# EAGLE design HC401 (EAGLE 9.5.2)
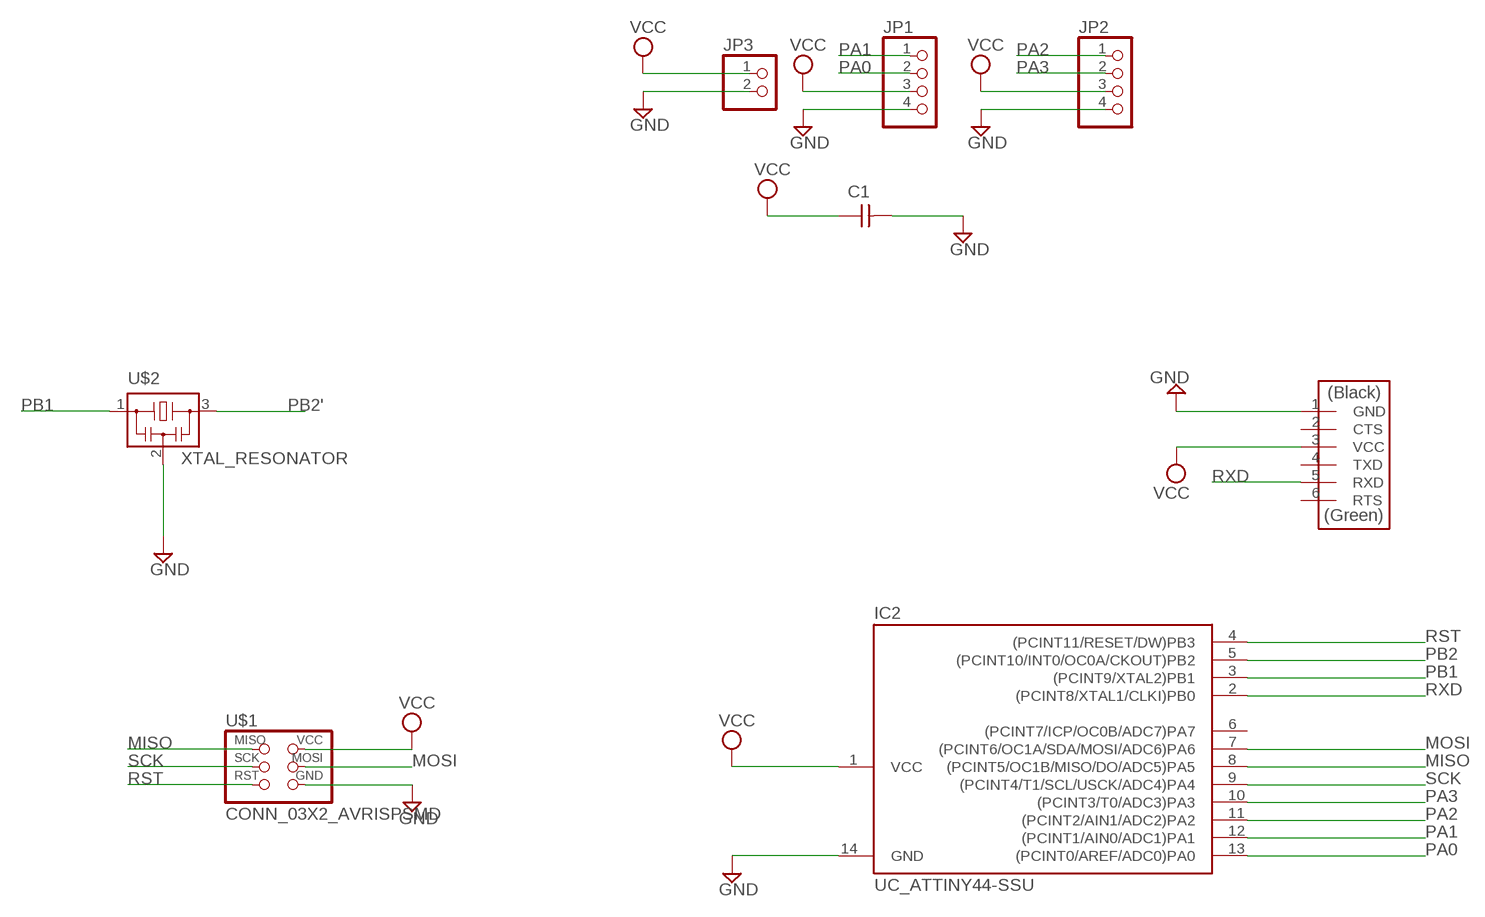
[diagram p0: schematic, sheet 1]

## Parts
C1  CAP_UNPOLARIZED  [C1206]
IC2  UC_ATTINY44-SSU  [SOIC14]
JP1  PINHD-1X4  [1X04]
JP2  PINHD-1X4  [1X04]
JP3  PINHD-1X2  [1X02]
U$1  CONN_03X2_AVRISPSMD  [2X03SMD]
U$2  XTAL_RESONATOR  [EFOBM]
U$3  CONN_06_FTDI-SMD-HEADER  [1X06SMD]

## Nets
GND: C1.2 IC2.14(GND) JP1.4 JP2.4 JP3.2 U$1.6(GND) U$2.2 U$3.1(GND)
MISO: IC2.8((PCINT5/OC1B/MISO/DO/ADC5)PA5) U$1.1(MISO)
MOSI: IC2.7((PCINT6/OC1A/SDA/MOSI/ADC6)PA6) U$1.4(MOSI)
PA0: IC2.13((PCINT0/AREF/ADC0)PA0) JP1.2
PA1: IC2.12((PCINT1/AIN0/ADC1)PA1) JP1.1
PA2: IC2.11((PCINT2/AIN1/ADC2)PA2) JP2.1
PA3: IC2.10((PCINT3/T0/ADC3)PA3) JP2.2
PB1: IC2.3((PCINT9/XTAL2)PB1) U$2.1
PB2: IC2.5((PCINT10/INT0/OC0A/CKOUT)PB2)
PB2': U$2.3
RST: IC2.4((PCINT11/RESET/DW)PB3) U$1.5(RST)
RXD: IC2.2((PCINT8/XTAL1/CLKI)PB0) U$3.5(RXD)
SCK: IC2.9((PCINT4/T1/SCL/USCK/ADC4)PA4) U$1.3(SCK)
VCC: C1.1 IC2.1(VCC) JP1.3 JP2.3 JP3.1 U$1.2(VCC) U$3.3(VCC)
Unconnected: IC2.6((PCINT7/ICP/OC0B/ADC7)PA7) U$3.2(CTS) U$3.4(TXD) U$3.6(RTS)

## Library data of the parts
C1 = fab:CAP_UNPOLARIZED
IC2 = fab:UC_ATTINY44
JP1 JP2 = pinhead:PINHD-1X4: PIN HEADER
JP3 = pinhead:PINHD-1X2: PIN HEADER
U$1 = fab:CONN_03X2_AVRISP
U$2 = fab:XTAL_RESONATOR
U$3 = fab:CONN_06_FTDI-SMD-HEADER

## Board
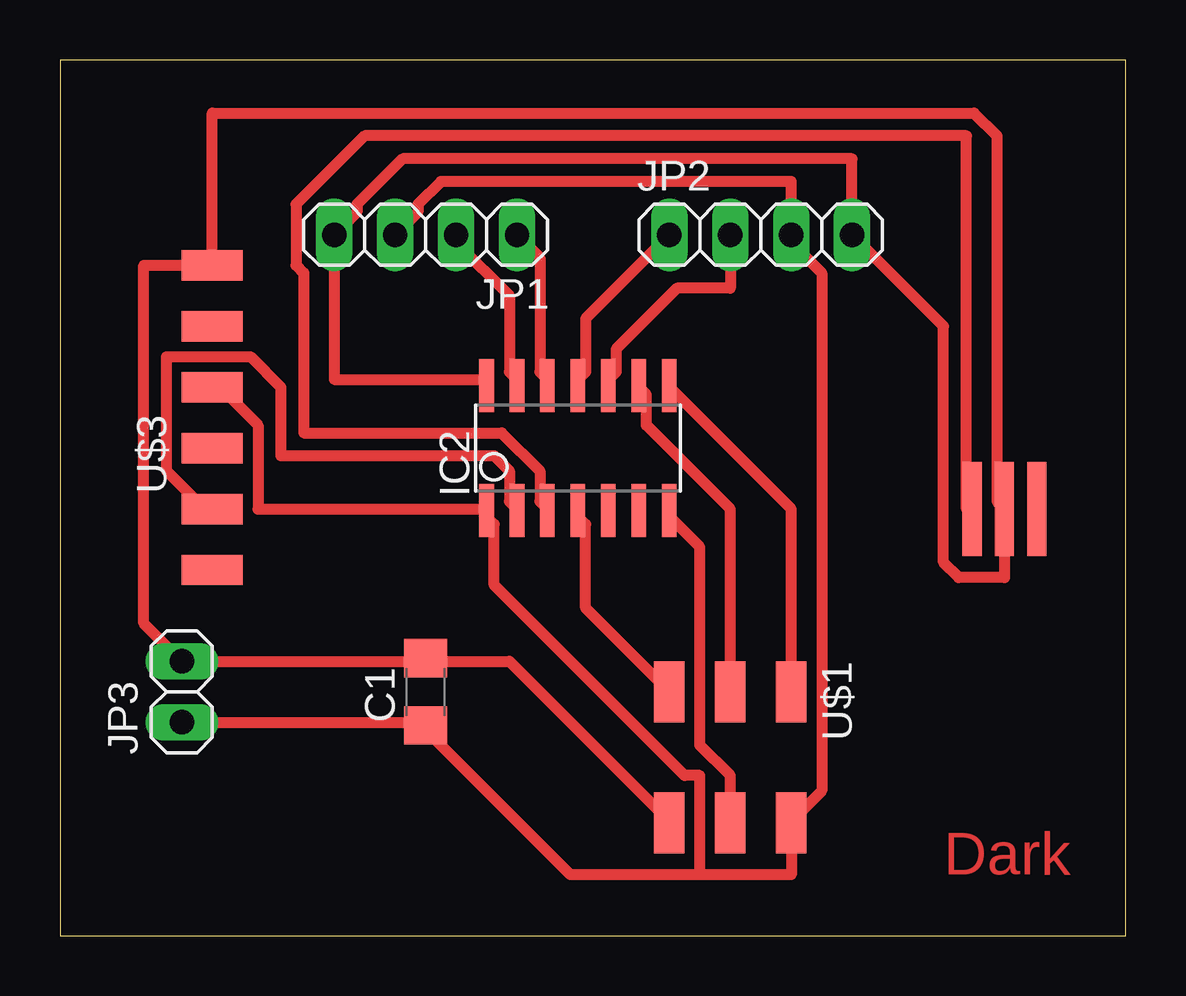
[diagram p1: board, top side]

Size 44.43 x 36.5 mm. Coordinates in mm from the lower left corner, seen from the top.
Outline: 0,0 44.43,0 44.43,36.5 0,36.5 0,0
Copper layers (1*16): Top 0.035mm / dielectric 1.5mm / Bottom 0.035mm
Design rules "fab-1": minimum track width 0.45mm, minimum drill 32mil, track to track 16mil, track to pad 16mil, pad to pad 16mil, via to via 16mil, smd to smd 6mil, copper to edge 16mil, drill to drill 16mil, minimum pad ring 10mil, minimum via ring 8mil, stop-mask expansion 4mil, vias tented up to drill 0mil, thermal gap 16mil

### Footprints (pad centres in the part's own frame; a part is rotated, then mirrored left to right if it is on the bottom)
C1206 = smd 1.6 x 1.8: 1 -1.4,0; 2 1.4,0
SOIC14 = smd 0.61 x 2.21: 1 -3.81,-2.603; 2 -2.54,-2.603; 3 -1.27,-2.603; 4 0,-2.603; 5 1.27,-2.603; 6 2.54,-2.603; 7 3.81,-2.603; 8 3.81,2.603; 9 2.54,2.603; 10 1.27,2.603; 11 0,2.603; 12 -1.27,2.603; 13 -2.54,2.603; 14 -3.81,2.603
1X04 = drill 1.016 long: 1 -3.81,0; 2 -1.27,0; 3 1.27,0; 4 3.81,0
1X02 = drill 1.016 long: 1 -1.27,0; 2 1.27,0
2X03SMD = smd 2.54 x 1.27: 1 -2.54,2.54; 2 2.92,2.54; 3 -2.54,0; 4 2.92,0; 5 -2.54,-2.54; 6 2.92,-2.54
EFOBM = smd 0.8 x 3.9: 1 -1.35,0; 2 0,0; 3 1.35,0
1X06SMD = smd 2.54 x 1.27: 1 0,6.35; 2 0,3.81; 3 0,1.27; 4 0,-1.27; 5 0,-3.81; 6 0,-6.35

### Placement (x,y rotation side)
C1  15.24,10.16 90 top
IC2  21.59,20.32 0 top
JP1  15.24,29.21 180 top
JP2  29.21,29.21 0 top
JP3  5.08,10.16 90 top
U$1  27.94,7.62 270 top
U$2  39.37,17.78 0 top
U$3  6.35,21.59 0 top

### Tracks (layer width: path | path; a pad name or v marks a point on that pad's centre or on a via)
GND
  Top 0.45: IC2.14 17.78,23.18 11.43,23.18 JP1.4 12.38,30.16 12.38,30.48 14.29,32.38 33.02,32.38 JP2.4 36.83,25.4 36.83,15.56 37.47,14.92 39.37,14.92 U$2.2 39.05,18.1 39.05,33.34 38.1,34.29 6.35,34.29 U$3.1 3.49,27.94 3.49,13.02 JP3.2 15.24,11.43 | 15.24,11.43 18.73,11.43 25.4,4.76 U$1.6 | 15.24,11.43 C1.2
MISO
  Top 0.45: U$1.1 30.48,17.78 25.4,22.86 IC2.8
MOSI
  Top 0.45: U$1.4 27.94,6.67 26.67,7.94 26.67,16.19 25.4,17.46 IC2.7
PA0
  Top 0.45: JP1.2 16.51,28.89 18.73,26.67 18.73,23.49 19.05,23.18 IC2.13
PA1
  Top 0.45: JP1.1 20,28.26 20,23.49 20.32,23.18 IC2.12
PA2
  Top 0.45: JP2.1 21.91,25.72 21.91,23.49 21.59,23.18 IC2.11
PA3
  Top 0.45: JP2.2 27.94,26.99 25.72,26.99 23.18,24.45 23.18,23.49 22.86,23.18 IC2.10
PB1
  Top 0.45: IC2.3 20.32,17.78 20,18.1 20,19.37 18.42,20.95 10.16,20.95 10.16,27.62 9.84,27.94 9.84,30.48 12.7,33.34 37.78,33.34 37.78,17.78 U$2.1
RST
  Top 0.45: U$1.5 21.91,13.65 21.91,17.14 21.59,17.46 IC2.4
RXD
  Top 0.45: U$3.5 6.03,17.78 4.45,19.37 4.45,24.13 7.94,24.13 9.21,22.86 9.21,20 18.1,20 18.73,19.37 18.73,18.1 19.05,17.78 IC2.2
SCK
  Top 0.45: U$1.3 27.94,17.78 24.45,21.27 24.45,22.54 24.13,22.86 IC2.9
VCC
  Top 0.45: U$3.3 6.67,22.86 8.26,21.27 8.26,17.78 17.78,17.78 IC2.1 17.78,17.46 18.1,17.14 18.1,14.6 26.04,6.67 26.67,6.67 26.67,2.54 | JP3.1 15.24,8.89 C1.1 15.24,8.57 21.27,2.54 26.67,2.54 | JP1.3 14.92,30.16 14.92,30.48 15.88,31.43 30.48,31.43 JP2.3 30.48,28.89 31.75,27.62 31.75,6.03 30.48,4.76 U$1.2 30.48,2.54 26.67,2.54

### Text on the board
Top: Dark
